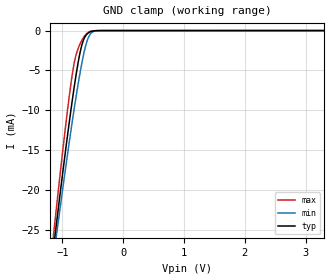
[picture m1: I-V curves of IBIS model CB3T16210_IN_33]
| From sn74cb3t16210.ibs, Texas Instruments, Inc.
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[Model]   CB3T16210_IN_33
Model_type  Input
Vinl=0.8
Vinh=2.0
| variable   typ   min   max
C_comp   2.59pF   2.00pF   3.29pF
[Temperature Range]   40   100   -40
| Ambient temperature   25   85   -40
[Voltage range]   3.3   3   3.6
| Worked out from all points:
|   GND clamp passes 1 mA (typ) near -0.64 V on its own axis
[GND Clamp]
| CB3T16210_IN_33
|   Voltage   I(typ)   I(min)   I(max)
-5.5V     -338.9mA   -314.3mA   -369mA
-1.14V    -26.82mA   -28.07mA   -25.13mA
-1.105V   -24.61mA   -26.05mA   -22.65mA
-1.075V   -22.73mA   -24.34mA   -20.55mA
-915mV    -13.07mA   -15.45mA   -9.893mA
-860mV    -9.954mA   -12.53mA   -6.658mA
-805mV    -7.019mA   -9.733mA   -4.027mA
-730mV    -3.528mA   -6.174mA   -2.02mA
-665mV    -1.428mA   -3.486mA   -1.009mA
-585mV    -362.1uA   -1.111mA   -263.9uA
-510mV    -78.77uA   -204.1uA   -38.82uA
3.3V      76.2pA     212.8pA    43.07pA
